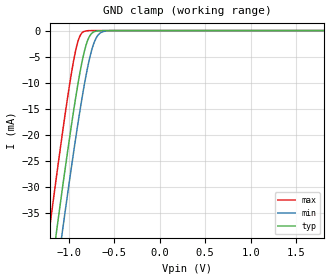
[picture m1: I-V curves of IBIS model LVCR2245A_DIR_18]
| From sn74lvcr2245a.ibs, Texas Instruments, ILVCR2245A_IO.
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[Model]   LVCR2245A_DIR_18
Model_type  Input
Vinl=0.5775
Vinh=1.2675
| variable   typ   min   max
C_comp   3.47pF   3.22pF   4.03pF
[Temperature Range]   40   100   -40
| Ambient temperature   25   85   -40
[Voltage range]   1.8   1.65   1.95
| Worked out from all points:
|   GND clamp passes 1 mA (typ) near -0.77 V on its own axis
[GND Clamp]
| LVCR2245A_DIR_18
|   Voltage   I(typ)   I(min)   I(max)
-5.5V     -655.9mA   -662.8mA   -647.2mA
-1.215V   -49.64mA   -57.94mA   -39mA
-1.135V   -39.11mA   -47.4mA    -28.45mA
-1.075V   -31.38mA   -39.64mA   -20.77mA
-1.055V   -28.84mA   -37.09mA   -18.29mA
-955mV    -16.69mA   -24.69mA   -6.88mA
-885mV    -9.107mA   -16.56mA   -1.487mA
-825mV    -3.926mA   -10.27mA   -137.3uA
-780mV    -1.473mA   -6.233mA   -17.16uA
-715mV    -205.6uA   -2.13mA    -809.3nA
-650mV    -22.03uA   -444.3uA   -37.97nA
1.8V      3.326pA    6.145pA    3.026pA
